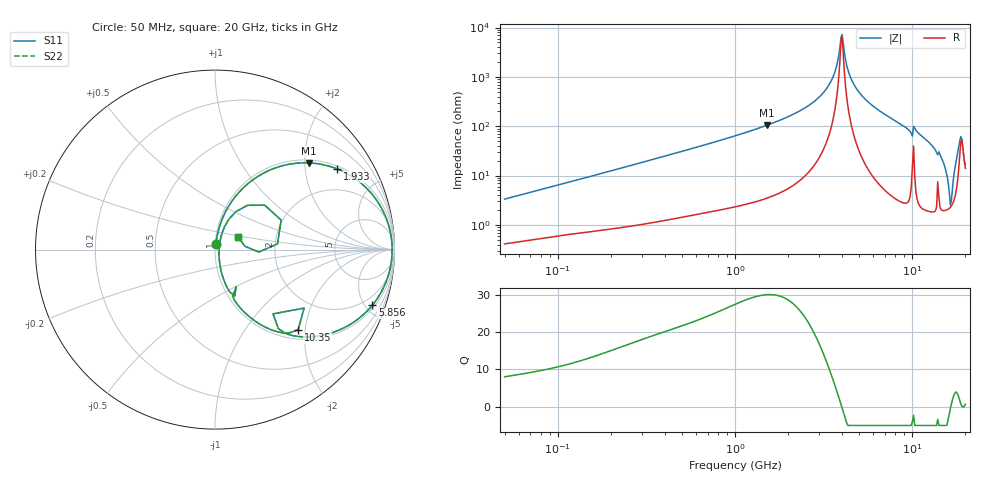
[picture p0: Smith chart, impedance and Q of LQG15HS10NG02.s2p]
!Murata Part Number: LQG15HS10NG02
!These Parameters are Measured in Series Mode Connection
!  o--[Z]--o
!Port1  Port2
!  o-------o
!Freq. Start=50[MHz] Stop=20[GHz], 401[Steps]
# Hz S RI R 50
!Freq.(Hz) S11(Real) S11(Imag) S21(Real) S21(Imag) S12(Real) S12(Imag) S22(Real) S22(Imag)
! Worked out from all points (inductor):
!   401 points, 50 MHz to 20 GHz, reference 50 ohm
!   read as one part in series: L = 10.4 nH near 51.52 MHz
!   highest Q = 30.1 at 1.521 GHz (marker M1), where L = 11 nH
!   self-resonance near 3.967 GHz
!   S11 on the Smith chart (normalised r, x): 50 MHz: 1.01, +0.07; 1.933 GHz: 1.10, +2.97; 5.856 GHz: 1.22, -5.56; 10.35 GHz: 1.20, -1.83; 20 GHz: 1.28, +0.19
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5e7  0.00519 0.0328  0.9948 -0.0328  0.9948 -0.0328  0.00519 0.0328
1.364002e8  0.0141 0.0843  0.9859 -0.0843  0.9859 -0.0843  0.0141 0.0843
3.721004e8  0.0601 0.2135  0.9399 -0.2135  0.9399 -0.2135  0.0601 0.2135
1e9  0.296 0.4387  0.704 -0.4387  0.704 -0.4387  0.296 0.4387
1.521052e9  0.5253 0.483  0.4747 -0.483  0.4747 -0.483  0.5253 0.483
1.932977e9  0.6822 0.4487  0.3178 -0.4487  0.3178 -0.4487  0.6822 0.4487
2.728004e9  0.8863 0.2943  0.1137 -0.2943  0.1137 -0.2943  0.8863 0.2943
3.466789e9  0.9713 0.1209  0.0287 -0.1209  0.0287 -0.1209  0.9713 0.1209
4.026975e9  0.987 -0.004  0.013 0.004  0.013 0.004  0.987 -0.004
4.34015e9  0.9824 -0.0683  0.0176 0.0683  0.0176 0.0683  0.9824 -0.0683
4.608136e9  0.9725 -0.1195  0.0275 0.1195  0.0275 0.1195  0.9725 -0.1195
5.856089e9  0.8762 -0.3104  0.1238 0.3104  0.1238 0.3104  0.8762 -0.3104
7.442007e9  0.695 -0.4469  0.305 0.4469  0.305 0.4469  0.695 -0.4469
9.745021e9  0.3872 -0.4638  0.6128 0.4638  0.6128 0.4638  0.3872 -0.4638
1.034674e10  0.4632 -0.4473  0.5368 0.4473  0.5368 0.4473  0.4632 -0.4473
1.238412e10  0.1967 -0.3783  0.8033 0.3783  0.8033 0.3783  0.1967 -0.3783
1.460232e10  0.0687 -0.2131  0.9313 0.2131  0.9313 0.2131  0.0687 -0.2131
1.646126e10  0.0225 -0.0101  0.9775 0.0101  0.9775 0.0101  0.0225 -0.0101
1.696185e10  0.0295 0.0546  0.9705 -0.0546  0.9705 -0.0546  0.0295 0.0546
1.774144e10  0.078 0.1701  0.922 -0.1701  0.922 -0.1701  0.078 0.1701
1.855685e10  0.2771 0.2476  0.7229 -0.2476  0.7229 -0.2476  0.2771 0.2476
2e10  0.1288 0.0713  0.8712 -0.0713  0.8712 -0.0713  0.1288 0.0713
